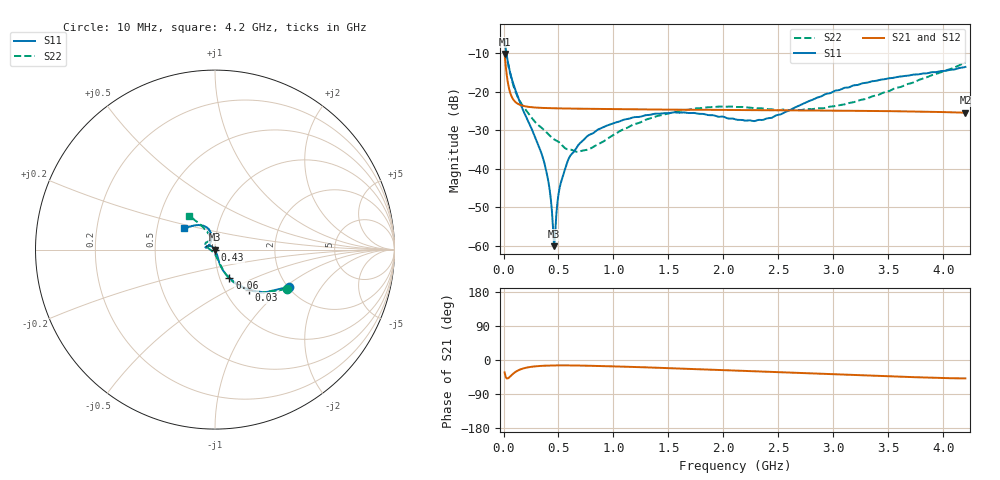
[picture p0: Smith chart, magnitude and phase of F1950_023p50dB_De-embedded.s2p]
! Integrated Device Technology
! Corporate Headquarters
! 6024 Silver Creek Valley Road
! San Jose, CA 95138  USA
! Phone:  1-408-284-8200
! Toll Free:  1-800-223-1366
! Webpage:  http://www.idt.com/
! Timing and RF Division
! 515 Groton Road, Suite 102
! Westford, MA 01886-6024
! Device:  F1950
! Description: 7-bit 0.25 dB Digital Step Attenuator
! Frequency:  150.0 -  4000.00 MHz
! Package:  4x4 mm Thin QFN Plastic Package: 24 pin
! Ports:  2 RF, 12 DC
!  Pin  1  = D0
!  Pin  2  = VDD
!  Pin  3  = Vmode
!  Pin  4  = GND
!  Pin  5  = RF1  =  Port 1
!  Pin  6  = GND
!  Pin  7  = GND
!  Pin  8  = GND
!  Pin  9  = GND
!  Pin 10  = GND
!  Pin 11  = GND
!  Pin 12  = GND
!  Pin 13  = GND
!  Pin 14  = RF2  =  Port 2
!  Pin 15  = GND
!  Pin 16  = LE
!  Pin 17  = CLK
!  Pin 18  = DATE
!  Pin 19  = D6
!  Pin 20  = D5
!  Pin 21  = D4
!  Pin 22  = D3
!  Pin 23  = D2
!  Pin 24  = D1
! State:  94
! Atten State:  23.50 dB
! Voltage:  +5.00 Volts
! Current:  Not Measured mA
! Data:  The device was measured on a the F195X evaluation board which has
!  individual transmission lines to the RF pins.  Data was collected
!  using a calibrated network analyzer.  The evaluation board was
!  de-embedded using a TRL calibration technique.
!  The reference plane is the edge of the package pin.
! Misc:  Board 2019
!  Action Tracker AT0250
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# GHz S dB R 50
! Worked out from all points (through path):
!   420 points, 10 MHz to 4.2 GHz, reference 50 ohm
!   highest |S21| = -10.23 dB at 10 MHz (marker M1); lowest = -25.4 dB at 4.2 GHz (marker M2)
!   group delay of S21, straight-line fit = 22.5 ps
!   lowest |S11| = -60.1 dB at 460 MHz (marker M3), VSWR 1.00, Z = 49.9 - j0.0596 ohm
!   |S11| at or under -10 dB: 26.57 MHz to end of sweep
!   |S22| runs from -35.6 to -6.8 dB; largest |S21 - S12| = 0.00011
!   S11 on the Smith chart (normalised r, x): 10 MHz: 2.04, -1.07; 30 MHz: 1.29, -0.63; 60 MHz: 1.11, -0.36; 430 MHz: 1.00, -0.01; 4.2 GHz: 0.69, +0.17
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0.01  -6.69 -26.5  -10.23 -32.8  -10.23 -32.8  -6.83 -29.0
0.03  -10.64 -49.7  -15.77 -48.8  -15.77 -48.8  -11.03 -51.9
0.06  -15.01 -62.9  -20.20 -43.6  -20.20 -43.6  -15.25 -64.2
0.1  -18.88 -69.8  -22.42 -33.2  -22.42 -33.2  -19.28 -69.3
0.15  -22.82 -71.7  -23.40 -25.2  -23.39 -25.2  -22.48 -73.3
0.35  -36.41 -67.6  -24.19 -15.4  -24.19 -15.4  -29.42 -83.0
0.4  -42.08 -69.7  -24.24 -14.8  -24.24 -14.8  -30.78 -84.7
0.43  -47.83 -78.2  -24.27 -14.5  -24.27 -14.5  -31.64 -87.6
0.45  -55.21 -97.6  -24.29 -14.4  -24.28 -14.4  -32.15 -90.8
0.46  -60.07 -143.0  -24.29 -14.3  -24.29 -14.4  -32.35 -92.6
0.48  -51.97 143.4  -24.30 -14.3  -24.30 -14.3  -32.67 -95.4
0.51  -44.94 135.8  -24.32 -14.2  -24.32 -14.2  -33.20 -98.2
0.56  -40.06 132.6  -24.34 -14.2  -24.34 -14.2  -34.64 -105.9
0.61  -36.49 134.5  -24.37 -14.3  -24.37 -14.3  -35.01 -117.2
0.71  -32.98 136.4  -24.40 -14.7  -24.40 -14.8  -35.32 -137.7
0.99  -28.25 146.5  -24.50 -16.8  -24.50 -16.7  -31.38 -179.9
1.41  -25.69 162.4  -24.62 -20.5  -24.61 -20.6  -26.21 160.5
2.11  -27.18 157.0  -24.75 -27.9  -24.74 -28.0  -23.95 142.3
2.43  -26.83 124.9  -24.80 -31.2  -24.80 -31.2  -24.53 131.5
2.81  -22.09 104.4  -24.86 -35.6  -24.86 -35.6  -24.51 116.0
3.51  -16.49 116.8  -25.03 -43.2  -25.02 -43.2  -19.79 113.1
4.2  -13.56 145.5  -25.44 -48.6  -25.44 -48.7  -12.48 127.1
